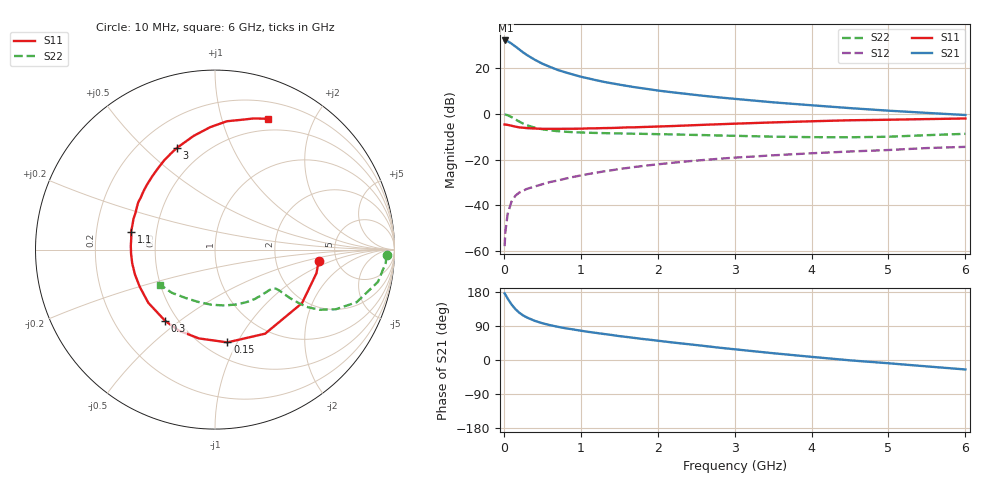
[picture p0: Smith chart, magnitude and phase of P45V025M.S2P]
! SIEMENS Small Signal Semiconductors
! BFP182
! Si NPN RF Bipolar Junction Transistor in SOT143
! VCE = 5 V  IC = 25 mA
! Common Emitter S-Parameters:  March  1996
# GHz  S  MA  R  50
!  f  S11  S21  S12  S22
! GHz  MAG  ANG  MAG  ANG  MAG  ANG  MAG  ANG
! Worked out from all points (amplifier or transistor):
!   36 points, 10 MHz to 6 GHz, reference 50 ohm
!   highest |S21| = 31.9 dB at 20 MHz (marker M1)
!   |S21| within 3 dB of that: start of sweep to 165.2 MHz
!   unconditionally stable (mu >= 1): 702.4 MHz to 5.435 GHz
!   at 250 MHz: K = 0.53, MSG = 30.1 dB, |S12| = -33.6 dB
!   at 1.4 GHz: K = 1.17, MAG = 16.5 dB, |S12| = -24.7 dB
!   at 6 GHz: K = 0.94, MSG = 6.9 dB, |S12| = -14.5 dB
!   S11 on the Smith chart (normalised r, x): 10 MHz: 3.64, -0.69; 150 MHz: 0.64, -0.91; 300 MHz: 0.43, -0.44; 1.1 GHz: 0.36, +0.09; 3 GHz: 0.35, +0.63; 6 GHz: 0.37, +1.41
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0.01  0.5814 -6.2  39.18 175.9  0.0013 94.6  0.9561 -1.9
0.02  0.5804 -13.1  39.33 172.7  0.0027 80.2  0.9543 -4.4
0.05  0.5692 -31.6  37.88 162.0  0.0066 79.9  0.9256 -11.2
0.1  0.5454 -59.2  33.52 146.6  0.0122 65.3  0.8416 -20.4
0.15  0.5215 -82.4  29.13 134.2  0.0163 60.1  0.7505 -26.3
0.2  0.5029 -100.3  25.13 124.9  0.0191 54.7  0.6723 -29.9
0.25  0.4944 -114.0  21.63 117.7  0.0209 53.3  0.6095 -31.8
0.3  0.4845 -124.9  18.97 112.2  0.023 52.0  0.5607 -32.5
0.4  0.4754 -141.4  15.03 103.5  0.0259 51.5  0.496 -32.9
0.5  0.4678 -153.6  12.29 97.1  0.029 51.3  0.4575 -32.7
0.6  0.467 -162.7  10.45 92.0  0.0324 52.9  0.4327 -32.5
0.7  0.4675 -170.6  8.965 87.7  0.035 54.2  0.4158 -32.5
0.8  0.4682 -177.0  7.947 83.8  0.0384 54.8  0.4041 -32.7
1  0.471 172.1  6.394 77.3  0.0451 55.1  0.3896 -33.8
1.1  0.4781 168.0  5.853 74.2  0.0485 55.6  0.384 -34.8
1.5  0.4937 152.3  4.294 63.1  0.0622 54.5  0.3718 -39.4
2.2  0.5382 130.3  2.908 46.1  0.0854 50.1  0.3536 -51.0
3  0.6052 110.5  2.105 28.3  0.1102 43.4  0.3297 -67.9
3.5  0.6448 100.6  1.768 17.9  0.1238 38.7  0.3156 -80.3
4.5  0.7182 84.7  1.321 -0.9  0.1501 30.1  0.3062 -107.8
5.5  0.7622 73.5  1.04 -16.9  0.1782 21.9  0.3402 -135.0
6  0.7856 68.1  0.935 -25.0  0.1893 17.0  0.364 -147.7
